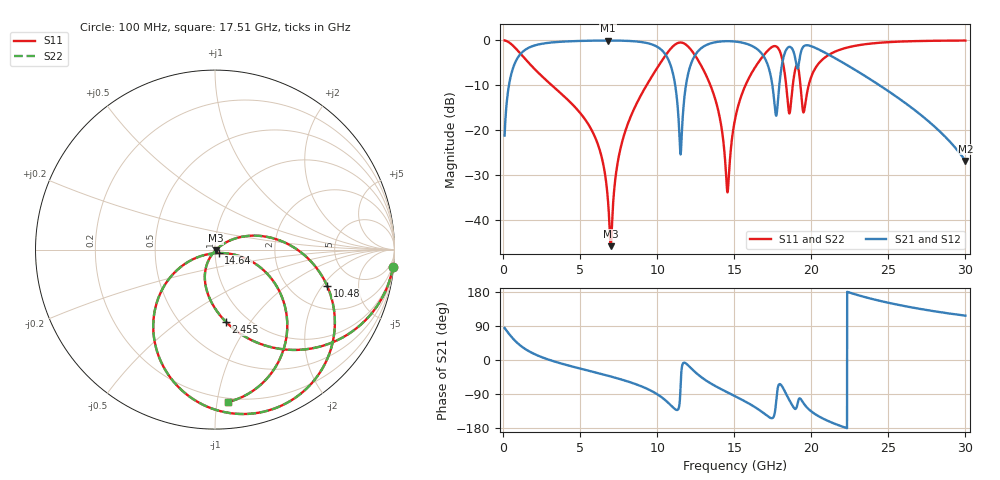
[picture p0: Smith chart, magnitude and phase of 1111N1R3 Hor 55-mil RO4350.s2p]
# GHz S MA R 50
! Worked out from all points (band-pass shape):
!   3201 points, 100 MHz to 30 GHz, reference 50 ohm
!   highest |S21| = -0.05 dB at 6.809 GHz (marker M1); lowest = -26.9 dB at 30 GHz (marker M2)
!   |S21| within 3 dB of the highest: 1.133 GHz to 10.51 GHz (9.379 GHz wide, 161 % of centre); 12.51 GHz to 16.8 GHz (4.292 GHz wide, 29.3 % of centre)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
!   lowest |S11| = -45.9 dB at 6.986 GHz (marker M3), VSWR 1.01, Z = 50.4 - j0.341 ohm
!   |S11| at or under -10 dB: 3.152 GHz to 9.317 GHz (6.164 GHz wide, 98.9 % of centre); 13.45 GHz to 15.73 GHz (2.281 GHz wide, 15.6 % of centre); 19.3 GHz to 19.83 GHz (537.8 MHz wide, 2.75 % of centre)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
!   |S22| runs from -45.9 to 0.0 dB; largest |S21 - S12| = 0
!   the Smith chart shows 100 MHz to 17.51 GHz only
!   S11 on the Smith chart (normalised r, x): 100 MHz: 1, -20; 2.455 GHz: 0.80, -0.77; 10.48 GHz: 3.14, -2.21; 14.64 GHz: 1.04, -0.04; 17.51 GHz: 0.17, -1.07
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0.1  0.9962 -5.6  0.08661 84.4  0.08661 84.4  0.9962 -5.6
0.7914375  0.8224 -39.7  0.568 50.2  0.568 50.2  0.8224 -39.7
2.454625  0.4078 -81.4  0.9109 8.4  0.9109 8.4  0.4078 -81.4
5.089563  0.1484 -112.3  0.9851 -23.5  0.9851 -23.5  0.1484 -112.3
6.808813  0.01625 -114.2  0.9943 -41.5  0.9943 -41.5  0.01625 -114.2
6.986344  0.005062 -42.0  0.9941 -43.5  0.9941 -43.5  0.005062 -42.0
7.845969  0.08721 32.2  0.9887 -53.5  0.9887 -53.5  0.08721 32.2
10.06978  0.5135 -4.8  0.8329 -92.1  0.8329 -92.1  0.5135 -4.8
10.48091  0.6558 -17.8  0.7157 -104.4  0.7157 -104.4  0.6558 -17.8
11.51806  0.9454 -69.2  0.05337 -70.3  0.05337 -70.3  0.9454 -69.2
12.36834  0.7151 -113.5  0.6399 -28.3  0.6399 -28.3  0.7151 -113.5
13.78859  0.2145 -153.1  0.9531 -69.1  0.9531 -69.1  0.2145 -153.1
14.63888  0.02854 -41.9  0.9781 -87.0  0.9781 -87.0  0.02854 -41.9
15.05  0.1308 -14.6  0.9691 -95.4  0.9691 -95.4  0.1308 -14.6
16.65713  0.5965 -47.6  0.752 -132.8  0.752 -132.8  0.5965 -47.6
17.50741  0.8522 -85.1  0.2868 -152.5  0.2868 -152.5  0.8522 -85.1
18.06803  0.6626 -129.5  0.4989 -67.3  0.4989 -67.3  0.6626 -129.5
18.57259  0.1528 -107.0  0.8452 -105.6  0.8452 -105.6  0.1528 -107.0
19.03044  0.5186 -88.6  0.5373 -126.7  0.5373 -126.7  0.5186 -88.6
20.03956  0.4089 -55.0  0.8543 -136.9  0.8543 -136.9  0.4089 -55.0
25.01978  0.9542 -120.4  0.2697 150.9  0.2697 150.9  0.9542 -120.4
30  0.994 -155.2  0.04528 117.1  0.04528 117.1  0.994 -155.2
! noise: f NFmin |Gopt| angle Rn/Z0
0.1  0.00245  0.9345  2.502  0.008331
3.417  0.01265  0.5742  24.5  0.005162
6.743  0.02441  0.5717  42.22  0.009075
10.06  0.07045  0.7597  59.81  0.04492
13.39  0.08002  0.728  80.37  0.03477
16.7  0.1406  0.8023  95.3  0.06796
20.03  0.1493  0.7803  112  0.04499
23.35  0.1514  0.7711  123.9  0.03161
26.67  0.2792  0.8702  139.4  0.05764
30  0.8855  0.9584  156.2  0.2075
